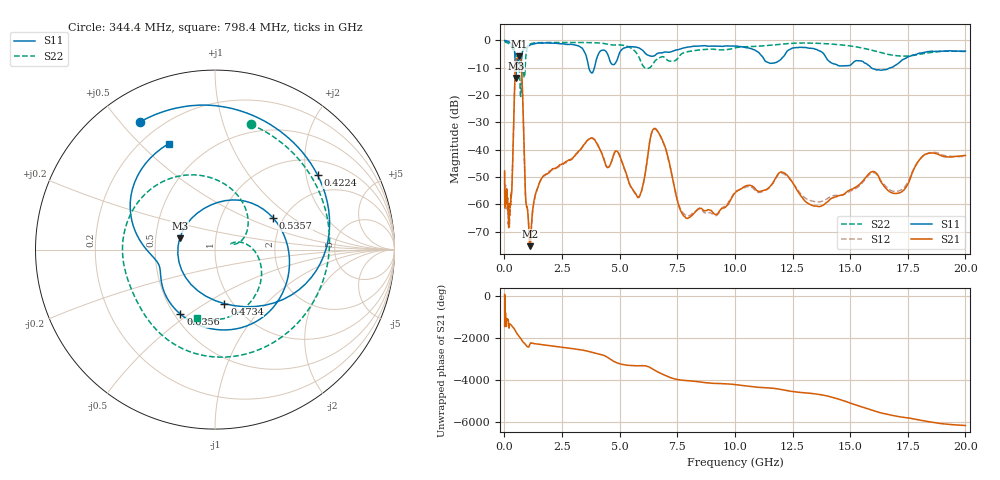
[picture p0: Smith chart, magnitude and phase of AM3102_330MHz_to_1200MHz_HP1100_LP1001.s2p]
! Date/Time: Tue, Sep 11, 2018 5:21 PM
! Network Analyzer: Agilent Technologies E8362B Rev: A.07.50.63
! Sweep from 0.010 to 20.000 GHz, 1601 Points, Sweep Type: LOG
! Power Supply: 4.949 V, 0.001 A
# Hz S DB R 50
!freq MagS11 AngS11 MagS21 AngS21 MagS12 AngS12 MagS22 AngS22
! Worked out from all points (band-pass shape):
!   1601 points, 10 MHz to 20 GHz, reference 50 ohm
!   highest |S21| = -5.75 dB at 647.8 MHz (marker M1); lowest = -75.2 dB at 1.119 GHz (marker M2)
!   |S21| within 3 dB of the highest: 486.2 MHz to 729.4 MHz (243.2 MHz wide, 40 % of centre)
!   lowest |S11| = -13.7 dB at 496.5 MHz (marker M3), VSWR 1.52, Z = 33.3 + j4.43 ohm
!   |S11| at or under -10 dB: 472.5 MHz to 522.7 MHz (50.2 MHz wide, 10.1 % of centre); 3.663 GHz to 3.906 GHz (242.8 MHz wide, 6.42 % of centre); 15.91 GHz to 16.76 GHz (846.9 MHz wide, 5.18 % of centre)
!   |S22| runs from -20.5 to -0.2 dB; largest |S21 - S12| = 0.0096
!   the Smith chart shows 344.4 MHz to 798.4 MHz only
!   S11 on the Smith chart (normalised r, x): 344.4 MHz: 0.13, +0.57; 422.4 MHz: 1.40, +2.33; 473.4 MHz: 0.92, -0.61; 535.7 MHz: 1.77, +0.72; 635.6 MHz: 0.54, -0.46; 798.4 MHz: 0.30, +0.61
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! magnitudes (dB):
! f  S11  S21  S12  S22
! 10 MHz  0.0  -47.7  -48.2  -0.2
! 35.55 MHz  -0.1  -58.4  -61.4  -0.4
! 126.4 MHz  -0.3  -58.1  -61.7  -0.9
! 184.8 MHz  -0.5  -67.7  -66.4  -1.1
! 344.4 MHz  -1.7  -49.3  -49.5  -2.8
! 422.4 MHz  -3.0  -23.5  -23.6  -4.2
! 447.2 MHz  -4.5  -16.4  -16.5  -4.4
! 473.4 MHz  -10.3  -10.6  -10.6  -5.1
! 496.5 MHz  -13.7  -7.8  -7.9  -5.7
! 535.7 MHz  -8.7  -6.7  -6.7  -5.8
! 635.6 MHz  -7.8  -5.8  -5.8  -9.4
! 647.8 MHz  -8.3  -5.8  -5.8  -10.8
! 709 MHz  -9.5  -7.1  -7.1  -20.4
! 798.4 MHz  -3.8  -21.9  -22.0  -8.1
! 920.7 MHz  -2.8  -57.3  -57.8  -6.8
! 1.119 GHz  -1.7  -75.2  -73.7  -1.3
! 1.59 GHz  -1.0  -50.8  -51.0  -0.8
! 3.775 GHz  -11.8  -35.7  -35.6  -0.8
! 5.652 GHz  -2.4  -55.5  -55.8  -3.8
! 6.549 GHz  -5.4  -32.3  -32.4  -7.4
! 7.958 GHz  -2.5  -65.1  -64.2  -4.1
! 20 GHz  -3.9  -42.1  -42.6  -4.1
